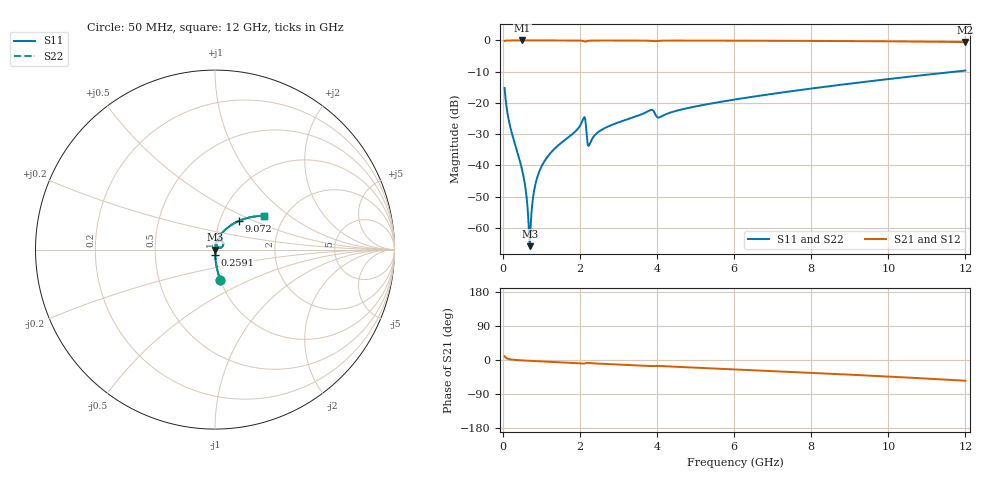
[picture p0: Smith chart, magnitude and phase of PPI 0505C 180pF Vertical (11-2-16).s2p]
# GHz S MA R 50
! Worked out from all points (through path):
!   1601 points, 50 MHz to 12 GHz, reference 50 ohm
!   highest |S21| = 0.00 dB at 513.1 MHz (marker M1); lowest = -0.5 dB at 12 GHz (marker M2)
!   group delay of S21, straight-line fit = 12.7 ps
!   lowest |S11| = -65.8 dB at 699.8 MHz (marker M3), VSWR 1.00, Z = 50.1 - j0.00193 ohm
!   |S11| at or under -10 dB: start of sweep to 11.72 GHz
!   |S22| runs from -65.8 to -9.6 dB; largest |S21 - S12| = 0
!   S11 on the Smith chart (normalised r, x): 50 MHz: 1.00, -0.35; 259.1 MHz: 1.00, -0.06; 9.072 GHz: 1.23, +0.41; 12 GHz: 1.57, +0.66
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0.05  0.173 -80.1  0.9847 9.8  0.9847 9.8  0.173 -80.1
0.1620312  0.05152 -87.2  0.9984 2.5  0.9984 2.5  0.05152 -87.2
0.259125  0.02942 -88.4  0.9992 0.9  0.9992 0.9  0.02942 -88.4
0.5130625  0.008007 -87.9  0.9995 -1.1  0.9995 -1.1  0.008007 -87.9
0.5952188  0.004155 -85.0  0.9995 -1.6  0.9995 -1.6  0.004155 -85.0
0.6624375  0.001482 -72.2  0.9995 -1.9  0.9995 -1.9  0.001482 -72.2
0.6997813  0.0005108 -2.2  0.9994 -2.1  0.9994 -2.1  0.0005108 -2.2
0.737125  0.001424 66.2  0.9994 -2.3  0.9994 -2.3  0.001424 66.2
0.796875  0.00337 78.2  0.9994 -2.6  0.9994 -2.6  0.00337 78.2
0.8491562  0.00501 80.8  0.9994 -2.9  0.9994 -2.9  0.00501 80.8
1.020938  0.009982 82.9  0.9993 -3.7  0.9993 -3.7  0.009982 82.9
2.044156  0.04778 72.0  0.9912 -8.9  0.9912 -8.9  0.04778 72.0
2.111375  0.05901 52.2  0.9705 -9.4  0.9705 -9.4  0.05901 52.2
2.253281  0.0218 61.0  0.9918 -8.0  0.9918 -8.0  0.0218 61.0
2.611781  0.03855 77.5  0.9975 -10.2  0.9975 -10.2  0.03855 77.5
3.806781  0.07563 67.1  0.9877 -15.9  0.9877 -15.9  0.07563 67.1
4.038312  0.05835 61.8  0.9853 -15.5  0.9853 -15.5  0.05835 61.8
6.025  0.1136 64.5  0.9916 -24.7  0.9916 -24.7  0.1136 64.5
8.019156  0.1705 55.5  0.9831 -33.9  0.9831 -33.9  0.1705 55.5
9.07225  0.2059 50.5  0.9761 -39.0  0.9761 -39.0  0.2059 50.5
10.01331  0.2414 45.7  0.9677 -43.8  0.9677 -43.8  0.2414 45.7
12  0.3295 34.9  0.9408 -54.6  0.9408 -54.6  0.3295 34.9
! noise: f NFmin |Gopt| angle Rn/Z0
0.05  0.0003251  0.8399  0.3064  0.00043
1.372  0.003201  0.6098  4.049  0.001518
2.701  0.006323  0.6115  7.936  0.003006
4.031  0.02352  0.8242  12.18  0.02779
5.36  0.009464  0.5188  14.98  0.003387
6.682  0.01079  0.4882  18.1  0.003535
8.012  0.01247  0.4774  21.18  0.003939
9.341  0.01432  0.4755  24.18  0.004461
10.67  0.01636  0.4803  27.11  0.005107
12  0.01863  0.4908  30  0.005909
